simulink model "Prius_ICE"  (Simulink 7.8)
settings: Solver=ode23tb  StartTime=0.0  StopTime=1180  RelTol=1e-3
InitFcn:
  | init_Prius_GT
StopFcn:
  | Vyhodnoceni
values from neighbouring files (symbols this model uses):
  om_diff_ic = 0    [init_Prius_GT.m]
  omric = 0    [init_Prius_GT.m]
  rpm_FMEP = [1,500,1000,1500,2000,2500,3000,3500,4000,4500,5000]    [init_Prius_GT.m]
  t_sample = 0.1    [init_Prius_GT.m]
  torque_FMEP = [0,0,0.58,0.66,0.75,0.84,0.93,1.1,1.3,1.4,1.5].*(Vdis/(4*pi))*100000    [init_Prius_GT.m]
  vf0 = 0    [init_Prius_GT.m]
undefined symbols (not defined in the file or in its folder): Clutch, Control, Differential, Driveshaft, Engine, Environment, Gearbox, Powertrain, table_FMEP, Vehicle
libraries: simulink x30, simulink_extras x6, simulink_need_slupdate x1
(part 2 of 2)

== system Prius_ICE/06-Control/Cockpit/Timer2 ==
  Set : Inport
  Add1 : Sum  Inputs=-+
  Clock : Clock
  Memory : Memory
  Switch1 : Switch  Threshold=1
  Count : Outport
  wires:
  Switch1/1 -> Memory/1
  Memory/1 -> Add1/1, Switch1/1
  Clock/1 -> Add1/2, Switch1/3
  Add1/1 -> Count/1
  Set/1 -> Switch1/2

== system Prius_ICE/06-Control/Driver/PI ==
  In1 : Inport
  Add3 : Sum  Inputs=+-
  Constant : Constant  Value=0.8
  Integrator1 : Integrator
  Product1 : Product
  Out1 : Outport
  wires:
  Add3/1 -> Product1/1
  Product1/1 -> Integrator1/1
  In1/1 -> Add3/1
  Integrator1/1 -> Add3/2, Out1/1
  Constant/1 -> Product1/2

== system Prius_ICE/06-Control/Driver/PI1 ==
  In1 : Inport
  Add3 : Sum  Inputs=+-
  Constant : Constant
  Integrator1 : Integrator
  Product1 : Product
  Out1 : Outport
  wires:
  Constant/1 -> Product1/2
  Integrator1/1 -> Out1/1, Add3/2
  In1/1 -> Add3/1
  Product1/1 -> Integrator1/1
  Add3/1 -> Product1/1

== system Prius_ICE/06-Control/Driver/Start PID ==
  Throttle : Inport
  n_eng[rpm] : Inport  Port=2
  StatusNum[-] : Inport  Port=3
  Add : Sum
  Add3 : Sum  Inputs=+-
  Constant2 : Constant  Value=0
  PID Controller : simulink/Continuous/PID Controller  Controller=PID  TimeDomain=Continuous-time  SampleTime=1  IntegratorMethod=Forward Euler  FilterMethod=Forward Euler  Form=Parallel  P=0.001  I=0.00001  D=0  N=100  InitialConditionSource=internal  InitialConditionForIntegrator=0  InitialConditionForFilter=0  ExternalReset=rising  LimitOutput=on  UpperSaturationLimit=1  LowerSaturationLimit=0  LinearizeAsGain=off  AntiWindupMode=none  Kb=1  TrackingMode=off  Kt=1  PParamMin=[]  PParamMax=[]  IParamMin=[]  IParamMax=[]  DParamMin=[]  DParamMax=[]  NParamMin=[]  NParamMax=[]  KbParamMin=[]  KbParamMax=[]  KtParamMin=[]  KtParamMax=[]  POutMin=[]  POutMax=[]  IOutMin=[]  IOutMax=[]  DOutMin=[]  DOutMax=[]  NOutMin=[]  NOutMax=[]  KbOutMin=[]  KbOutMax=[]  KtOutMin=[]  KtOutMax=[]  IntegratorOutMin=[]  IntegratorOutMax=[]  FilterOutMin=[]  FilterOutMax=[]  SumOutMin=[]  SumOutMax=[]  SumI1OutMin=[]  SumI1OutMax=[]  SumI2OutMin=[]  SumI2OutMax=[]  SumI3OutMin=[]  SumI3OutMax=[]  SumDOutMin=[]  SumDOutMax=[]  SaturationOutMin=[]  SaturationOutMax=[]  IntegratorContinuousStateAttributes=''  IntegratorStateMustResolveToSignalObject=off  IntegratorRTWStateStorageClass=Auto  FilterContinuousStateAttributes=''  FilterStateMustResolveToSignalObject=off  FilterRTWStateStorageClass=Auto
  Scope : Scope  NumInputPorts=4
  Start rpm : Constant  Value=Engine.Idle.rpm*2.5
  Switch : Switch  Threshold=1
  Te_dem : Outport
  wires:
  Add/1 -> Scope/1, Te_dem/1
  n_eng[rpm]/1 -> Add3/2, Scope/3
  Constant2/1 -> Switch/3
  Switch/1 -> Add/2, Scope/2
  Add3/1 -> PID Controller/1
  Start rpm/1 -> Add3/1
  PID Controller/1 -> Switch/1
  Throttle/1 -> Add/1
  StatusNum[-]/1 -> Scope/4, Switch/2, PID Controller/2

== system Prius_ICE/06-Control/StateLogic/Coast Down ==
  Gear : Inport
  v_veh : Inport  Port=2
  Compare To Constant3 : simulink/Logic and Bit Operations/Compare To Constant  relop===  const=0  OutDataTypeStr=uint8
  Compare To Constant4 : simulink/Logic and Bit Operations/Compare To Constant  relop=<=  const=1  OutDataTypeStr=boolean
  Detect Decrease1 : simulink/Logic and Bit Operations/Detect Decrease  vinit=0.0  InputProcessing=Inherited  OutDataTypeStr=uint8
  Logical Operator4 : Logic  AllPortsSameDT=off  OutDataTypeStr=boolean
  S-R Flip-Flop2 : simulink_extras/Flip Flops/S-R Flip-Flop  initial_condition=0
  Terminator : Terminator
  Roll off : Outport
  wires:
  Detect Decrease1/1 -> Logical Operator4/2
  Compare To Constant3/1 -> Logical Operator4/1
  Logical Operator4/1 -> S-R Flip-Flop2/1
  Compare To Constant4/1 -> S-R Flip-Flop2/2
  S-R Flip-Flop2/1 -> Roll off/1
  Gear/1 -> Compare To Constant3/1, Detect Decrease1/1
  v_veh/1 -> Compare To Constant4/1
  S-R Flip-Flop2/2 -> Terminator/1

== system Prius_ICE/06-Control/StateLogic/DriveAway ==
  Gear : Inport
  ClutchLocked : Inport  Port=2
  Compare To Constant : simulink/Logic and Bit Operations/Compare To Constant  relop===  const=1  OutDataTypeStr=uint8
  Detect Increase : simulink/Logic and Bit Operations/Detect Increase  vinit=0.0  InputProcessing=Inherited  OutDataTypeStr=uint8
  Logical Operator : Logic  AllPortsSameDT=off  OutDataTypeStr=boolean
  S-R Flip-Flop : simulink_extras/Flip Flops/S-R Flip-Flop  initial_condition=0
  Terminator : Terminator
  Drive away : Outport
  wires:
  Detect Increase/1 -> Logical Operator/2
  Compare To Constant/1 -> Logical Operator/1
  Logical Operator/1 -> S-R Flip-Flop/1
  S-R Flip-Flop/1 -> Drive away/1
  S-R Flip-Flop/2 -> Terminator/1
  Gear/1 -> Compare To Constant/1, Detect Increase/1
  ClutchLocked/1 -> S-R Flip-Flop/2

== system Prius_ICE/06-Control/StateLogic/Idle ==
  Gear : Inport
  v_veh : Inport  Port=2
  Drive_away : Inport  Port=3
  Compare To Constant3 : simulink/Logic and Bit Operations/Compare To Constant  relop===  const=0  OutDataTypeStr=uint8
  Compare To Constant4 : simulink/Logic and Bit Operations/Compare To Constant  relop=<=  const=1  OutDataTypeStr=boolean
  Logical Operator4 : Logic  AllPortsSameDT=off  OutDataTypeStr=boolean
  S-R Flip-Flop2 : simulink_extras/Flip Flops/S-R Flip-Flop  initial_condition=0
  Terminator : Terminator
  Idle : Outport
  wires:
  S-R Flip-Flop2/2 -> Terminator/1
  v_veh/1 -> Compare To Constant4/1
  Gear/1 -> Compare To Constant3/1
  S-R Flip-Flop2/1 -> Idle/1
  Logical Operator4/1 -> S-R Flip-Flop2/1
  Compare To Constant3/1 -> Logical Operator4/1
  Compare To Constant4/1 -> Logical Operator4/2
  Drive_away/1 -> S-R Flip-Flop2/2

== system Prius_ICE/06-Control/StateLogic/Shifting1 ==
  Gear : Inport
  ClutchLocked : Inport  Port=2
  Compare To Constant1 : simulink/Logic and Bit Operations/Compare To Constant  relop=~=  const=1  OutDataTypeStr=uint8
  Compare To Constant2 : simulink/Logic and Bit Operations/Compare To Constant  relop=~=  const=0  OutDataTypeStr=uint8
  Detect Decrease : simulink/Logic and Bit Operations/Detect Decrease  vinit=0.0  InputProcessing=Inherited  OutDataTypeStr=uint8
  Detect Increase1 : simulink/Logic and Bit Operations/Detect Increase  vinit=0.0  InputProcessing=Inherited  OutDataTypeStr=uint8
  Logical Operator1 : Logic  Inputs=3  AllPortsSameDT=off  OutDataTypeStr=boolean
  Logical Operator2 : Logic  AllPortsSameDT=off  OutDataTypeStr=boolean
  Logical Operator3 : Logic  Operator=OR  AllPortsSameDT=off  OutDataTypeStr=boolean
  S-R Flip-Flop1 : simulink_extras/Flip Flops/S-R Flip-Flop  initial_condition=0
  Terminator1 : Terminator
  Shifting : Outport
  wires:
  Detect Increase1/1 -> Logical Operator1/2
  Compare To Constant1/1 -> Logical Operator1/1
  Compare To Constant2/1 -> Logical Operator2/1
  Detect Decrease/1 -> Logical Operator2/2
  Logical Operator1/1 -> Logical Operator3/1
  Logical Operator2/1 -> Logical Operator3/2
  Logical Operator3/1 -> S-R Flip-Flop1/1
  S-R Flip-Flop1/1 -> Shifting/1
  S-R Flip-Flop1/2 -> Terminator1/1
  Gear/1 -> Compare To Constant1/1, Detect Increase1/1, Detect Decrease/1, Compare To Constant2/1
  ClutchLocked/1 -> S-R Flip-Flop1/2
